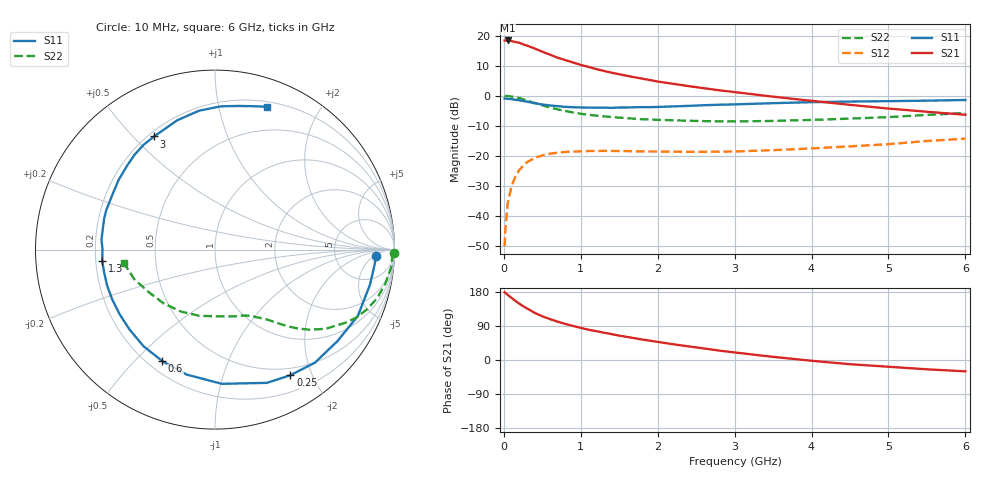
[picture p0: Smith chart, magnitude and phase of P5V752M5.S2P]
! SIEMENS Small Signal Semiconductors
! BFP183
! Si NPN RF Bipolar Junction Transistor in SOT143
! VCE = 0.75 V  IC = 2.5 mA
! Common Emitter S-Parameters:  March  1996
# GHz  S  MA  R  50
!  f  S11  S21  S12  S22
! GHz  MAG  ANG  MAG  ANG  MAG  ANG  MAG  ANG
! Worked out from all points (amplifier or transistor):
!   36 points, 10 MHz to 6 GHz, reference 50 ohm
!   highest |S21| = 18.4 dB at 50 MHz (marker M1)
!   |S21| within 3 dB of that: start of sweep to 430.3 MHz
!   unconditionally stable (mu >= 1): 1.853 GHz to end of sweep
!   at 250 MHz: K = 0.14, MSG = 20.3 dB, |S12| = -23.4 dB
!   at 1.4 GHz: K = 0.78, MSG = 13.0 dB, |S12| = -18.4 dB
!   at 6 GHz: K = 1.11, MAG = 1.9 dB, |S12| = -14.3 dB
!   S11 on the Smith chart (normalised r, x): 10 MHz: 16, -6; 250 MHz: 0.40, -1.70; 600 MHz: 0.26, -0.60; 1.3 GHz: 0.23, -0.05; 3 GHz: 0.22, +0.58; 6 GHz: 0.25, +1.40
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0.01  0.8954 -2.3  8.325 178.7  0.0031 88.7  0.9961 -1.2
0.02  0.8939 -5.0  8.273 177.3  0.0061 85.5  0.9884 -2.2
0.05  0.8855 -12.7  8.332 171.9  0.0162 83.9  0.9873 -5.6
0.1  0.8775 -24.9  8.124 163.9  0.0308 76.2  0.9678 -11.3
0.15  0.8517 -36.8  7.863 156.1  0.0448 69.2  0.9441 -16.5
0.2  0.8408 -48.5  7.631 148.7  0.0574 63.3  0.9106 -21.4
0.25  0.8164 -59.0  7.182 142.0  0.0678 58.0  0.8727 -25.8
0.3  0.7969 -68.7  6.847 136.3  0.0777 53.3  0.834 -29.2
0.4  0.7488 -87.1  6.126 124.6  0.0914 44.4  0.7581 -35.6
0.5  0.7139 -102.8  5.406 115.3  0.1009 37.6  0.69 -40.3
0.6  0.6873 -115.3  4.831 107.9  0.1079 32.3  0.6359 -43.7
0.7  0.6694 -126.6  4.301 101.1  0.1123 28.1  0.5916 -46.3
0.8  0.6518 -136.9  3.918 95.1  0.1154 24.4  0.5555 -48.5
1.1  0.6337 -161.6  3.021 80.0  0.1195 17.1  0.4802 -53.9
1.3  0.632 -174.2  2.586 72.1  0.1201 13.7  0.4518 -57.0
1.7  0.6414 164.3  2.028 57.5  0.118 10.4  0.4126 -63.3
2.2  0.6626 144.1  1.577 41.6  0.1165 9.0  0.3894 -72.5
3  0.7159 118.3  1.148 19.9  0.1175 11.4  0.372 -91.2
3.5  0.7506 106.3  0.963 8.3  0.1235 13.4  0.3793 -104.2
4.5  0.7986 87.8  0.704 -11.1  0.1429 15.3  0.415 -134.1
5.5  0.8263 75.2  0.54 -24.6  0.1757 14.2  0.4783 -159.7
6  0.8475 69.9  0.481 -29.9  0.1922 10.9  0.513 -171.5
